| TEXAS INSTRUMENTS INCORPORATED
| Standard Linear and Logic Group
| IBIS Model of SN74LVCC4245A
| OCTAL DUAL-SUPPLY BUS TRANSCEIVER
| WITH CONFIGURABLE OUTPUT VOLTAGE AND 3-STATE OUTPUTS
| This file contains package information for the following:
|  TSSOP 24-pin (PW) package as [Component] LVCC4245A_PW
|  SSOP 24-pin (DB) package as [Component] LVCC4245A_DB
|  SOP 24-pin (NS) package as [Component] LVCC4245A_NS
|  SOIC 24-pin (DW) package as [Component] LVCC4245A_DW
| This device can be powered at the following Vccs:
|B-port
|3.3 volt Vcc
|5 volt Vcc
|A-port
|5 volt Vcc
|This file provides unique models under the [Model Selector] for each Vcc.
|For operation at a specific Vcc, select the appropriate model after each
|[Model Selector] keyword.
[IBIS Ver]   3.2
[Comment char]  |_char
[File Name]   sn74lvcc4245a.ibs
[File Rev]   1.1 | a_die
[Date]   October 29, 2002
[Source]   Data created from TI-SPICE simulations at TI-SLL.
[Notes]   The following is an IBIS list for the LVCC4245A.
   Please contact sllibis@ti.com with questions and
   comments concerning SLL IBIS models.
   - Due to the fact that the device is 5-V input/output
   tolerant, the pullup data has some non-monotonic warnings.
   - As there is no power clamp diode in the OE and DIR
   Models, we removed the Pwr Clamp table data from those
   Models.
[Disclaimer] Property of Texas Instruments Incorporated.  Unauthorized
   reproduction and/or distribution is strictly prohibited.
   This product is protected under copyright law.
   Created  2002, (C) Copyright  2002, Texas Instruments
   Incorporated, All Rights Reserved
   UNLESS THERE IS A SIGNED, WRITTEN AGREEMENT TO THE
   CONTRARY, TEXAS INSTRUMENTS (TI) IS PROVIDING THE IBIS
   MODELS  AND WITHOUT ANY WARRANTY, EXPRESSED OR
   IMPLIED.  TI assumes no liability for:
   1) the accuracy of the IBIS models provided to your
   company;
   2) the proper functioning of these IBIS Models in your
   design or for any resulting applications; or
   3) infringement of patents, copyrights or intellectual
   property rights resulting from your use of these IBIS
   models.
   TI provides IBIS Models as a service to our customers.
   You and your company shall not distribute, sell or give
   these models to anyone else without prior written
   permission from TI.
   TI reserves the right to make changes to our products or
   to discontinue any semiconductor product or service
   without notice, and advises our customers to obtain the
   latest version of relevant information to verify, before
   placing orders, that the information being relied on is
   current.
   Please be aware that your receipt and use of the IBIS
   information provided shall serve as acceptance of these
   terms and conditions.  If you do not accept these terms,
   you should return or destroy the IBIS models and any
   other accompanying information immediately.
| Component LVCC4245A_PW 24-pin TSSOP
[Component]   LVCC4245A_PW
[Manufacturer]   Texas Instruments, Inc.
[Package]
|   typ   min   max
R_pkg   3.900e-02   3.000e-02   4.600e-02
L_pkg   2.685e-09   2.367e-09   3.177e-09
C_pkg   3.200e-13   2.520e-13   4.340e-13
[Pin]   signal_name   model_name   R_pin   L_pin   C_pin
1   VCCA   POWER   3.700e-02   3.153e-09   4.340e-13
2   DIR   LVCC4245A_DIR   3.400e-02   2.629e-09   3.410e-13
3   A1   LVCC4245A_A   3.200e-02   2.860e-09   3.470e-13
4   A2   LVCC4245A_A   4.200e-02   2.741e-09   2.900e-13
5   A3   LVCC4245A_A   4.600e-02   2.600e-09   2.620e-13
6   A4   LVCC4245A_A   4.300e-02   2.414e-09   2.660e-13
7   A5   LVCC4245A_A   4.200e-02   2.367e-09   2.620e-13
8   A6   LVCC4245A_A   4.400e-02   2.461e-09   2.520e-13
9   A7   LVCC4245A_A   4.200e-02   2.543e-09   2.740e-13
10   A8   LVCC4245A_A   3.000e-02   2.616e-09   3.320e-13
11   GND   GND   3.700e-02   2.670e-09   3.460e-13
12   GND   GND   3.900e-02   3.177e-09   4.330e-13
13   GND   GND   3.700e-02   3.111e-09   4.310e-13
14   B8   LVCC4245A_B   3.700e-02   2.656e-09   3.450e-13
15   B7   LVCC4245A_B   3.100e-02   2.739e-09   3.400e-13
16   B6   LVCC4245A_B   4.200e-02   2.649e-09   2.820e-13
17   B5   LVCC4245A_B   4.600e-02   2.532e-09   2.570e-13
18   B4   LVCC4245A_B   4.400e-02   2.425e-09   2.660e-13
19   B3   LVCC4245A_B   4.400e-02   2.425e-09   2.660e-13
20   B2   LVCC4245A_B   4.600e-02   2.532e-09   2.570e-13
21   B1   LVCC4245A_B   4.200e-02   2.648e-09   2.820e-13
22   NOE   LVCC4245A_OE   3.100e-02   2.738e-09   3.390e-13
23   NC   NC   3.600e-02   2.653e-09   3.440e-13
24   VCCB   POWER   3.700e-02   3.110e-09   4.310e-13
| Component LVCC4245A_DB 24-pin SSOP
[Component]   LVCC4245A_DB
[Manufacturer]   Texas Instruments, Inc.
[Package]
|   typ   min   max
R_pkg   4.500e-02   4.000e-02   4.900e-02
L_pkg   3.668e-09   3.226e-09   4.415e-09
C_pkg   4.160e-13   3.490e-13   5.070e-13
[Pin]   signal_name   model_name   R_pin   L_pin   C_pin
1   VCCA   POWER   4.200e-02   4.299e-09   5.030e-13
2   DIR   LVCC4245A_DIR   4.000e-02   3.960e-09   4.990e-13
3   A1   LVCC4245A_A   4.200e-02   3.775e-09   4.170e-13
4   A2   LVCC4245A_A   4.700e-02   3.487e-09   3.690e-13
5   A3   LVCC4245A_A   4.600e-02   3.347e-09   3.520e-13
6   A4   LVCC4245A_A   4.900e-02   3.352e-09   3.710e-13
7   A5   LVCC4245A_A   4.600e-02   3.226e-09   3.630e-13
8   A6   LVCC4245A_A   4.700e-02   3.289e-09   3.490e-13
9   A7   LVCC4245A_A   4.700e-02   3.347e-09   3.610e-13
10   A8   LVCC4245A_A   4.100e-02   3.576e-09   4.090e-13
11   GND   GND   4.100e-02   3.995e-09   5.030e-13
12   GND   GND   4.500e-02   4.415e-09   5.070e-13
13   GND   GND   4.300e-02   4.337e-09   5.060e-13
14   B8   LVCC4245A_B   4.200e-02   4.003e-09   5.040e-13
15   B7   LVCC4245A_B   4.100e-02   3.686e-09   4.100e-13
16   B6   LVCC4245A_B   4.800e-02   3.355e-09   3.490e-13
17   B5   LVCC4245A_B   4.700e-02   3.301e-09   3.530e-13
18   B4   LVCC4245A_B   4.800e-02   3.268e-09   3.660e-13
19   B3   LVCC4245A_B   4.800e-02   3.269e-09   3.660e-13
20   B2   LVCC4245A_B   4.700e-02   3.314e-09   3.490e-13
21   B1   LVCC4245A_B   4.800e-02   3.399e-09   3.550e-13
22   NOE   LVCC4245A_OE   4.100e-02   3.688e-09   4.120e-13
23   NC   NC   4.200e-02   4.003e-09   5.040e-13
24   VCCB   POWER   4.300e-02   4.347e-09   5.050e-13
| Component LVCC4245A_NS 24-pin SOP
[Component]   LVCC4245A_NS
[Manufacturer]   Texas Instruments, Inc.
[Package]
|   typ   min   max
R_pkg   4.400e-02   3.800e-02   4.800e-02
L_pkg   3.840e-09   2.545e-09   5.234e-09
C_pkg   5.860e-13   2.740e-13   7.970e-13
[Pin]   signal_name   model_name   R_pin   L_pin   C_pin
1   VCCA   POWER   4.100e-02   5.146e-09   7.650e-13
2   DIR   LVCC4245A_DIR   4.100e-02   4.357e-09   7.490e-13
3   A1   LVCC4245A_A   4.000e-02   3.923e-09   6.330e-13
4   A2   LVCC4245A_A   4.400e-02   3.412e-09   5.370e-13
5   A3   LVCC4245A_A   4.500e-02   3.036e-09   3.970e-13
6   A4   LVCC4245A_A   4.500e-02   2.845e-09   4.150e-13
7   A5   LVCC4245A_A   4.400e-02   2.843e-09   4.150e-13
8   A6   LVCC4245A_A   4.500e-02   3.065e-09   3.990e-13
9   A7   LVCC4245A_A   4.500e-02   3.529e-09   5.440e-13
10   A8   LVCC4245A_A   4.100e-02   4.013e-09   6.390e-13
11   GND   GND   4.100e-02   4.358e-09   7.460e-13
12   GND   GND   4.400e-02   5.234e-09   7.670e-13
13   GND   GND   3.900e-02   5.181e-09   7.650e-13
14   B8   LVCC4245A_B   4.800e-02   4.582e-09   7.640e-13
15   B7   LVCC4245A_B   4.100e-02   4.163e-09   6.550e-13
16   B6   LVCC4245A_B   4.600e-02   3.613e-09   5.490e-13
17   B5   LVCC4245A_B   4.700e-02   3.163e-09   4.060e-13
18   B4   LVCC4245A_B   4.700e-02   2.963e-09   4.220e-13
19   B3   LVCC4245A_B   4.700e-02   2.919e-09   4.190e-13
20   B2   LVCC4245A_B   4.800e-02   3.087e-09   4.870e-13
21   B1   LVCC4245A_B   4.600e-02   4.513e-09   7.600e-13
22   NOE   LVCC4245A_OE   4.200e-02   4.505e-09   7.670e-13
23   NC   NC   4.200e-02   5.163e-09   7.970e-13
24   VCCB   POWER   3.800e-02   2.545e-09   2.740e-13
| Component LVCC4245A_DW 24-pin SOIC
[Component]   LVCC4245A_DW
[Manufacturer]   Texas Instruments, Inc.
[Package]
|   typ   min   max
R_pkg   3.700e-02   3.000e-02   4.700e-02
L_pkg   5.146e-09   3.993e-09   6.885e-09
C_pkg   7.580e-13   5.120e-13   1.067e-12
[Pin]   signal_name   model_name   R_pin   L_pin   C_pin
1   VCCA   POWER   3.900e-02   6.885e-09   1.067e-12
2   DIR   LVCC4245A_DIR   4.200e-02   5.950e-09   9.580e-13
3   A1   LVCC4245A_A   4.700e-02   5.317e-09   7.910e-13
4   A2   LVCC4245A_A   3.100e-02   4.651e-09   6.110e-13
5   A3   LVCC4245A_A   3.000e-02   3.993e-09   5.120e-13
6   A4   LVCC4245A_A   3.000e-02   4.083e-09   6.110e-13
7   A5   LVCC4245A_A   3.000e-02   4.083e-09   6.110e-13
8   A6   LVCC4245A_A   3.000e-02   3.993e-09   5.120e-13
9   A7   LVCC4245A_A   3.100e-02   4.652e-09   6.110e-13
10   A8   LVCC4245A_A   4.700e-02   5.317e-09   7.910e-13
11   GND   GND   4.200e-02   5.950e-09   9.590e-13
12   GND   GND   3.900e-02   6.885e-09   1.067e-12
13   GND   GND   3.900e-02   6.885e-09   1.067e-12
14   B8   LVCC4245A_B   4.200e-02   5.950e-09   9.590e-13
15   B7   LVCC4245A_B   4.700e-02   5.317e-09   7.910e-13
16   B6   LVCC4245A_B   3.100e-02   4.652e-09   6.110e-13
17   B5   LVCC4245A_B   3.000e-02   3.993e-09   5.120e-13
18   B4   LVCC4245A_B   3.000e-02   4.083e-09   6.100e-13
19   B3   LVCC4245A_B   3.000e-02   4.083e-09   6.100e-13
20   B2   LVCC4245A_B   3.000e-02   3.993e-09   5.120e-13
21   B1   LVCC4245A_B   3.100e-02   4.651e-09   6.110e-13
22   NOE   LVCC4245A_OE   4.700e-02   5.317e-09   7.910e-13
23   NC   NC   4.200e-02   5.950e-09   9.580e-13
24   VCCB   POWER   3.900e-02   6.885e-09   1.067e-12
| Model LVCC4245A_DIR
[Model Selector]   LVCC4245A_DIR
LVCC4245A_DIR_33B   3.3 volt Vcc
LVCC4245A_DIR_50   5 volt Vcc
| Model LVCC4245A_OE
[Model Selector]   LVCC4245A_OE
LVCC4245A_OE_33B   3.3 volt Vcc
LVCC4245A_OE_50   5 volt Vcc
| Model LVCC4245A_B
[Model Selector]   LVCC4245A_B
LVCC4245A_B_33B   3.3 volt Vcc
LVCC4245A_B_50   5 volt Vcc
| Models and submodels in the file (7): LVCC4245A_DIR_33B (Input), LVCC4245A_DIR_50 (Input), LVCC4245A_OE_33B (Input), LVCC4245A_OE_50 (Input), LVCC4245A_A (I/O), LVCC4245A_B_33B (I/O), LVCC4245A_B_50 (I/O)
